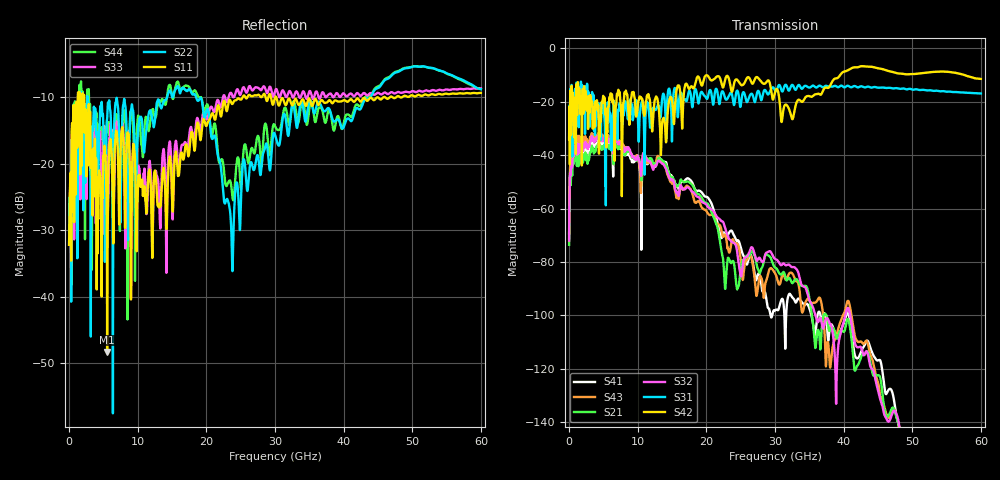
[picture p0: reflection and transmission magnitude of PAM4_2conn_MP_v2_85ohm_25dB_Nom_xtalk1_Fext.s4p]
! Info: Touchstone file created by Circ.  Input file=FAB50GbE_2conn_Midplane_Examax_Topo2_v2_85ohm_25dB_Nom.circ
# Hz S RI R 50
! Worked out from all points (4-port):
!   6000 points, 10 MHz to 60 GHz, reference 50 ohm
!   strongest paths, dB at 10 MHz, 15.01 GHz, 30.01 GHz, 45.01 GHz, 60 GHz:
!     S42: -34.0, -19.7, -16.3, -7.5, -11.4
!     S31: -33.9, -33.2, -15.8, -14.7, -16.9
!     S32: -72.0, -49.4, -78.8, -128.0, -168.5
!     S21: -73.5, -48.2, -82.0, -122.4, -161.6
!     S43: -71.2, -50.6, -84.2, -125.2, -170.7
!     S41: -69.3, -48.1, -98.2, -116.8, -173.3
!   lowest |S11| = -48.3 dB at 5.55 GHz (marker M1), VSWR 1.01, Z = 50.4 - j0.0304 ohm
!   |S11| at or under -10 dB: start of sweep to 1.277 GHz; 2.202 GHz to 25.31 GHz (23.11 GHz wide, 168 % of centre); 30.17 GHz to 45.88 GHz (15.71 GHz wide, 41.3 % of centre)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
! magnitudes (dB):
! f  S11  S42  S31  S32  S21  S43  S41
! 10 MHz  -32.2  -34.0  -33.9  -72.0  -73.5  -71.2  -69.3
! 810 MHz  -12.5  -25.8  -17.0  -36.6  -39.8  -33.7  -36.1
! 5.55 GHz  -48.3  -31.3  -28.0  -33.6  -35.8  -32.2  -35.0
! 25.33 GHz  -10.0  -13.7  -16.6  -80.6  -79.2  -86.7  -77.2
! 32.51 GHz  -11.3  -26.5  -13.7  -81.9  -87.9  -84.2  -93.2
! 41.45 GHz  -10.7  -7.1  -14.2  -107.7  -117.5  -105.2  -112.3
! 60 GHz  -9.4  -11.4  -16.9  -168.5  -161.6  -170.7  -173.3
